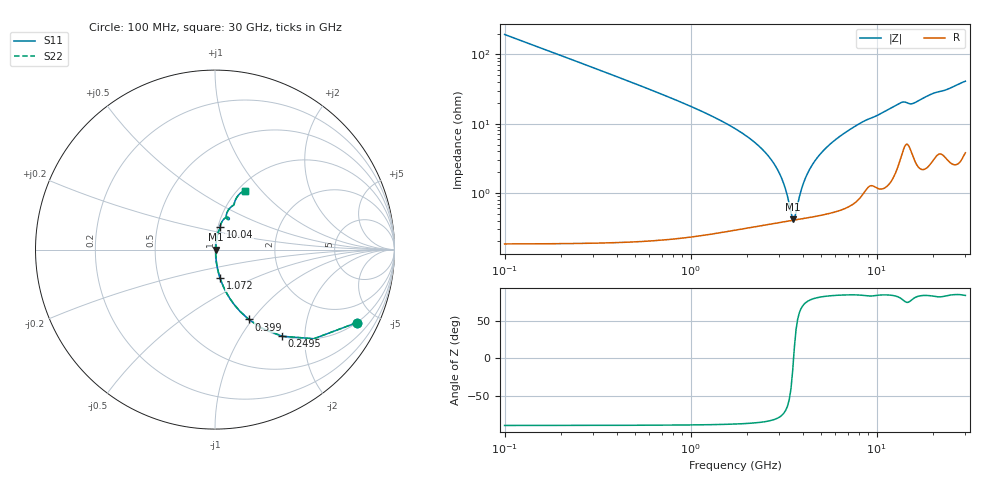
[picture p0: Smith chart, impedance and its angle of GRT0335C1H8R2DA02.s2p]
!Murata Part Number: GRT0335C1H8R2DA02
!These Parameters are Measured in Series Mode Connection
!Data Generated on Jun 19, 2026
!  o--ll--o
!Port1  Port2
!  o------o
!Operation Temp=25[degC], DC Bias Voltage=0[V]
!Freq. Start=100[MHz] Stop=30[GHz] 401[Steps]
# Hz S RI R 50
!Freq.(Hz) S11(Real) S11(Imag) S21(Real) S21(Imag) S12(Real) S12(Imag) S22(Real) S22(Imag)
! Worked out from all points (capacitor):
!   401 points, 100 MHz to 30 GHz, reference 50 ohm
!   read as one part in series: C = 8.2 pF near 249.5 MHz
!   lowest |Z| = 419 mohm at 3.538 GHz (marker M1)
!   series resonance near 3.576 GHz, so ESL is about 240 pH
!   S11 on the Smith chart (normalised r, x): 100 MHz: 1.00, -3.88; 249.5 MHz: 1.00, -1.55; 399 MHz: 1.00, -0.96; 1.072 GHz: 1.00, -0.33; 10.04 GHz: 1.02, +0.26; 30 GHz: 1.08, +0.82
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1e8  0.7897 -0.407  0.2103 0.407  0.2103 0.407  0.7897 -0.407
2.495e8  0.3749 -0.4829  0.6251 0.4829  0.6251 0.4829  0.3749 -0.4829
3.99e8  0.1883 -0.3889  0.8117 0.3889  0.8117 0.3889  0.1883 -0.3889
6.2325e8  0.0849 -0.2754  0.9151 0.2754  0.9151 0.2754  0.0849 -0.2754
1.07175e9  0.0284 -0.1592  0.9716 0.1592  0.9716 0.1592  0.0284 -0.1592
2.71625e9  0.00447 -0.0297  0.9955 0.0297  0.9955 0.0297  0.00447 -0.0297
3.09e9  0.00404 -0.0156  0.996 0.0156  0.996 0.0156  0.00404 -0.0156
3.46375e9  0.004 -0.00339  0.996 0.00339  0.996 0.00339  0.004 -0.00339
3.5385e9  0.00403 -0.00111  0.996 0.00111  0.996 0.00111  0.00403 -0.00111
3.688e9  0.00411 0.00329  0.9959 -0.00329  0.9959 -0.00329  0.00411 0.00329
3.987e9  0.00438 0.0116  0.9956 -0.0116  0.9956 -0.0116  0.00438 0.0116
4.286e9  0.00477 0.0194  0.9952 -0.0194  0.9952 -0.0194  0.00477 0.0194
5.10825e9  0.00631 0.0388  0.9937 -0.0388  0.9937 -0.0388  0.00631 0.0388
6.00525e9  0.00869 0.0578  0.9913 -0.0578  0.9913 -0.0578  0.00869 0.0578
7.1265e9  0.0128 0.0797  0.9872 -0.0797  0.9872 -0.0797  0.0128 0.0797
1.004175e10  0.0279 0.1256  0.9721 -0.1256  0.9721 -0.1256  0.0279 0.1256
1.01165e10  0.0281 0.1268  0.9719 -0.1268  0.9719 -0.1268  0.0281 0.1268
1.34055e10  0.064 0.1792  0.936 -0.1792  0.936 -0.1792  0.064 0.1792
1.505e10  0.0734 0.1673  0.9266 -0.1673  0.9266 -0.1673  0.0734 0.1673
2.005825e10  0.0916 0.2395  0.9084 -0.2395  0.9084 -0.2395  0.0916 0.2395
2.50665e10  0.1167 0.2827  0.8833 -0.2827  0.8833 -0.2827  0.1167 0.2827
3e10  0.1659 0.3283  0.8341 -0.3283  0.8341 -0.3283  0.1659 0.3283
